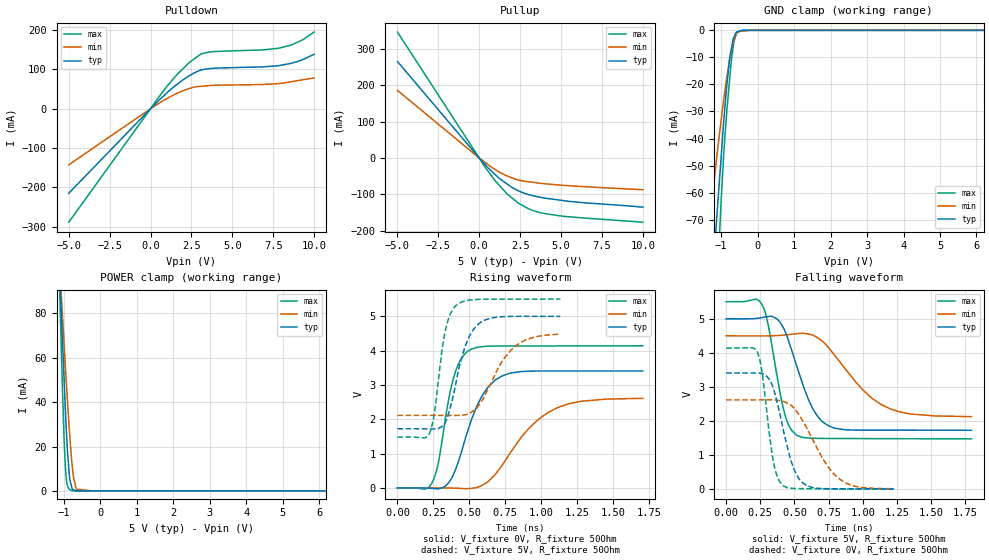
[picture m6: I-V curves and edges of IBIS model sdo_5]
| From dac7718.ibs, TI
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|   sdo_5 Model
[Model]   sdo_5
Model_type   3-state
Polarity   Non-Inverting
Vmeas = 2.5
Vref = 2.5
Cref = 5pF
Rref = 50
|   typ   min   max
|   (Nom PVT)   (Fast PVT)   (Slow PVT)
|C_comp from frequency method(F=50MHz)
|Average
|C_comp   3.377e-12   2.762e-12   3.961e-12
|   4.804e-12
|OFF state: BUFFER IN HIGH IMPEDANCE
|C_comp   3.952e-12   3.073e-12   4.804e-12
|ON state : BUFFER OUTPUT TURNED HIGH
|C_comp   3.405e-12   2.555e-12   4.167e-12
|C_comp from LC Tank Method (L=1nH)
|Resonant Frequency(Hz)   2.74e9   3.03e9   2.53e9
C_comp   3.377e-12   2.762e-12   3.961e-12
| Where nom  PVT is Nominal Process,  5V,  33C
|   Fast PVT is Strong Process,   5.5V,  -40C
|   Slow PVT is Weak Process,   4.5V,  113C
[Voltage Range]   5   4.5   5.5
|Ambient Temperature   25   85   -40
|Junction Temperature
[Temperature Range]   33   113   -40
[Pullup Reference]   5   4.5   5.5
[Pulldown Reference]   0   0   0
[Power Clamp Reference]   5   4.5   5.5
[GND Clamp Reference]   0   0   0
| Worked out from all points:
|   slope of the pulldown table from 0 to 0.75 V, typ, clamps not added: 24.4 ohm
|   slope of the pullup table from 0 to 0.75 V, typ, clamps not added: 20.8 ohm
|   GND clamp passes 1 mA (typ) near -0.60 V on its own axis
|   POWER clamp passes 1 mA (typ) near -0.77 V on its own axis
|   falling waveform, V_fixture 5V, R_fixture 50Ohm: 20-80 % time 174ps typ, 316ps min, 110ps max; typ from 5 V to 1.73 V
|   rising waveform, V_fixture 0V, R_fixture 50Ohm: 20-80 % time 179ps typ, 307ps min, 110ps max; typ from 0 V to 3.4 V
|   rising waveform, V_fixture 5V, R_fixture 50Ohm: 20-80 % time 122ps typ, 194ps min, 79.6ps max; typ from 1.72 V to 4.99 V
|   falling waveform, V_fixture 0V, R_fixture 50Ohm: 20-80 % time 126ps typ, 223ps min, 78.2ps max; typ from 3.41 V to 0.015 V
[Pulldown]
|   Voltage   I(typ)   I(min)   I(max)
-5V       -215.1mA   -142.7mA   -288.7mA
643.5mV   26.63mA    17.35mA    37.5mA
1.468V    57.19mA    36.17mA    79.84mA
2.376V    84.05mA    51.48mA    117.9mA
3.08V     98.28mA    56.96mA    139.2mA
3.547V    101.6mA    58.57mA    144.1mA
6.885V    106.5mA    61.59mA    149.7mA
7.821V    109.5mA    63.83mA    153.7mA
8.591V    115.4mA    68.61mA    161.9mA
9.3V      124.9mA    73.52mA    175.3mA
10V       138.4mA    78.36mA    194.9mA
[GND Clamp]
|   Voltage   I(typ)   I(min)   I(max)
-5V       -972.1mA   -679mA     -1.345A
-1.368V   -120mA     -78.23mA   -173.2mA
-1.228V   -90.84mA   -60.12mA   -129.8mA
-1.14V    -72.89mA   -49.33mA   -103.1mA
-1.083V   -62.35mA   -42.52mA   -86.24mA
-1.001V   -46.96mA   -33.27mA   -63.23mA
-907.5mV  -30.21mA   -23.49mA   -41.37mA
-765mV    -10.15mA   -10.67mA   -17.74mA
-654.5mV  -2.683mA   -3.922mA   -4.527mA
-585mV    -663.4uA   -1.309mA   -1.245mA
-202.5mV  -7.313uA   -80.45nA   -1.807uA
10V       0A         0A         0A
[Pullup]
|   Voltage   I(typ)   I(min)   I(max)
-5V       265.1mA    185.9mA    345.9mA
352mV     -17.79mA   -11.88mA   -24.5mA
973.5mV   -45.53mA   -31.6mA    -62.48mA
1.672V    -70.48mA   -48.4mA    -97.07mA
2.376V    -89.51mA   -60.05mA   -123.3mA
3.08V     -101.2mA   -65.42mA   -140.7mA
3.966V    -109.7mA   -70.38mA   -152.3mA
5.192V    -117.2mA   -75.01mA   -160.2mA
10V       -134.7mA   -87mA      -176.1mA
[POWER Clamp]
|   Voltage   I(typ)   I(min)   I(max)
-5V       341.3mA    268.4mA    345.5mA
-1.14V    108.2mA    108.6mA    106.5mA
-1.067V   79.58mA    87.61mA    62.52mA
-995.5mV  51.59mA    67.09mA    24.68mA
-946mV    32.21mA    52.89mA    7.951mA
-900mV    17.86mA    40.43mA    2.44mA
-840mV    5.417mA    25.41mA    602uA
-770mV    808.7uA    11.41mA    81.53uA
-742.5mV  596.2uA    7.017mA    35.34uA
-648mV    32.86uA    752.1uA    30.84uA
-202.5mV  12.12nA    0A         9.638uA
10V       0A         0A         0A
[Ramp]
R_load = 50
|   typ   min   max
dV/dt_r   2.04622/1.78826e-10   1.57181/3.0696e-10   2.48355/1.09089e-10
dV/dt_f   1.96473/1.74189e-10   1.42894/3.17689e-10   2.41171/1.10004e-10
[Falling Waveform]
V_fixture = 5V
V_fixture_min = 4.5V
V_fixture_max = 5.5V
R_fixture = 50Ohm
|   Time   V(typ)   V(min)   V(max)
0s        5V         4.5V       5.5V
264ps     5.037V     4.498V     5.405V
309ps     5.068V     4.5V       4.798V
425ps     4.688V     4.524V     2.271V
518ps     3.598V     4.564V     1.584V
636ps     2.351V     4.516V     1.499V
759ps     1.847V     4.109V     1.493V
1.005ns   1.738V     2.898V     1.49V
1.198ns   1.738V     2.364V     1.488V
1.795ns   1.733V     2.132V     1.483V
[Rising Waveform]
V_fixture = 0V
V_fixture_min = 0V
V_fixture_max = 0V
R_fixture = 50Ohm
|   Time   V(typ)   V(min)   V(max)
0s        2.196nV    2.837nV    1.899nV
241ps     -10.7mV    1.146mV    155.8mV
283ps     -25.13mV   1.272mV    701.1mV
390ps     393.4mV    -4.143mV   3.197V
509ps     1.915V     -12.83mV   4.027V
630ps     2.935V     183.3mV    4.124V
776ps     3.33V      969.4mV    4.131V
913ps     3.397V     1.727V     4.132V
1.115ns   3.403V     2.341V     4.133V
1.707ns   3.405V     2.609V     4.137V
[Rising Waveform]
V_fixture = 5V
V_fixture_min = 4.5V
V_fixture_max = 5.5V
R_fixture = 50Ohm
|   Time   V(typ)   V(min)   V(max)
0s        1.724V     2.113V     1.48V
221ps     1.719V     2.114V     1.57V
256ps     1.716V     2.114V     2.156V
330ps     1.887V     2.11V      4.509V
415ps     3.231V     2.112V     5.336V
491ps     4.329V     2.154V     5.461V
584ps     4.836V     2.511V     5.49V
719ps     4.982V     3.624V     5.494V
832ps     4.995V     4.165V     5.494V
1.133ns   4.994V     4.479V     5.497V
[Falling Waveform]
V_fixture = 0V
V_fixture_min = 0V
V_fixture_max = 0V
R_fixture = 50Ohm
|   Time   V(typ)   V(min)   V(max)
0s        3.411V     2.623V     4.138V
228ps     3.412V     2.624V     4.03V
263ps     3.391V     2.625V     3.425V
345ps     2.968V     2.623V     835.3mV
412ps     1.867V     2.59V      125mV
496ps     603.2mV    2.387V     29.7mV
589ps     110mV      1.808V     20.93mV
703ps     23.85mV    925.3mV    16.26mV
819ps     19.4mV     336.6mV    13.37mV
1.227ns   15.21mV    20.92mV    7.778mV
